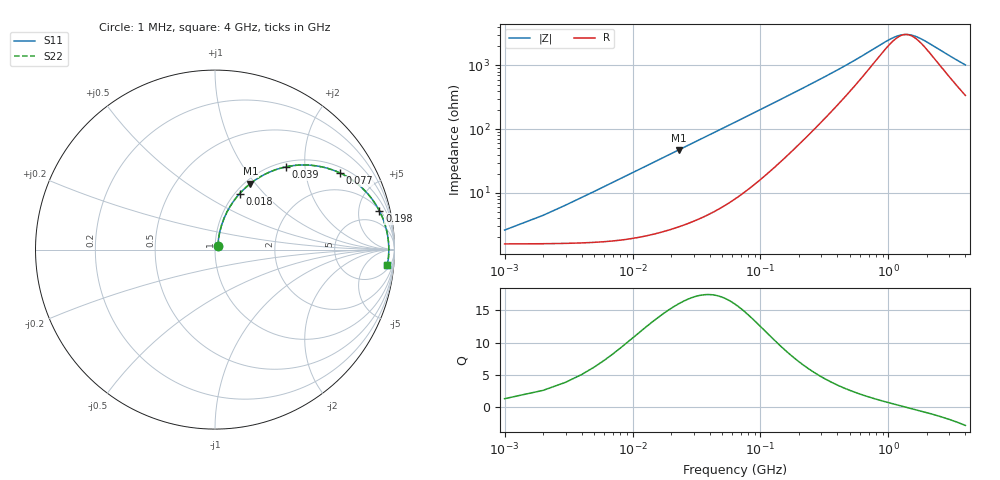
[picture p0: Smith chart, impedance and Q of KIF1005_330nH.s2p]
!version-2
!date-12.2020
!Series
# MHz S RI R 50
!Freq ReS11 ImS11 ReS21 ImS21 ReS12 ImS12 ReS22 ImS22
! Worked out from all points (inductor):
!   4000 points, 1 MHz to 4 GHz, reference 50 ohm
!   read as one part in series: L = 325 nH near 21 MHz
!   highest Q = 16 at 23 MHz (marker M1), where L = 326 nH
!   self-resonance near 1.372 GHz
!   S11 on the Smith chart (normalised r, x): 1 MHz: 1.03, +0.04; 18 MHz: 1.05, +0.74; 39 MHz: 1.09, +1.59; 77 MHz: 1.21, +3.12; 198 MHz: 2.13, +8.04; 4 GHz: 8, -19
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1  0.016 0.0201  0.984 -0.0201  0.984 -0.0201  0.016 0.0201
18  0.1371 0.3116  0.8629 -0.3116  0.8629 -0.3116  0.1371 0.3116
23  0.197 0.3678  0.803 -0.3678  0.803 -0.3678  0.197 0.3678
30  0.2849 0.423  0.7151 -0.423  0.7151 -0.423  0.2849 0.423
39  0.3936 0.4608  0.6064 -0.4608  0.6064 -0.4608  0.3936 0.4608
58  0.5774 0.4645  0.4226 -0.4645  0.4226 -0.4645  0.5774 0.4645
77  0.698 0.4262  0.302 -0.4262  0.302 -0.4262  0.698 0.4262
98  0.7813 0.3758  0.2187 -0.3758  0.2187 -0.3758  0.7813 0.3758
123  0.8408 0.3223  0.1592 -0.3223  0.1592 -0.3223  0.8408 0.3223
198  0.9159 0.2159  0.0841 -0.2159  0.0841 -0.2159  0.9159 0.2159
283  0.9431 0.1523  0.0569 -0.1523  0.0569 -0.1523  0.9431 0.1523
387  0.9557 0.1085  0.0443 -0.1085  0.0443 -0.1085  0.9557 0.1085
668  0.9654 0.0527  0.0346 -0.0527  0.0346 -0.0527  0.9654 0.0527
850  0.9672 0.0335  0.0328 -0.0335  0.0328 -0.0335  0.9672 0.0335
1022  0.9679 0.0201  0.0321 -0.0201  0.0321 -0.0201  0.9679 0.0201
1179  0.9683 0.0102  0.0317 -0.0102  0.0317 -0.0102  0.9683 0.0102
1334  0.9684 0.00187  0.0316 -0.00187  0.0316 -0.00187  0.9684 0.00187
1584  0.9683 -0.00974  0.0317 0.00974  0.0317 0.00974  0.9683 -0.00974
2001  0.9677 -0.0261  0.0323 0.0261  0.0323 0.0261  0.9677 -0.0261
2667  0.966 -0.0481  0.034 0.0481  0.034 0.0481  0.966 -0.0481
3334  0.9637 -0.0678  0.0363 0.0678  0.0363 0.0678  0.9637 -0.0678
4000  0.9607 -0.0861  0.0393 0.0861  0.0393 0.0861  0.9607 -0.0861
